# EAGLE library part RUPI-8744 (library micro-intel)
MICROCOMPUTER/PERIPHERAL DEVICE
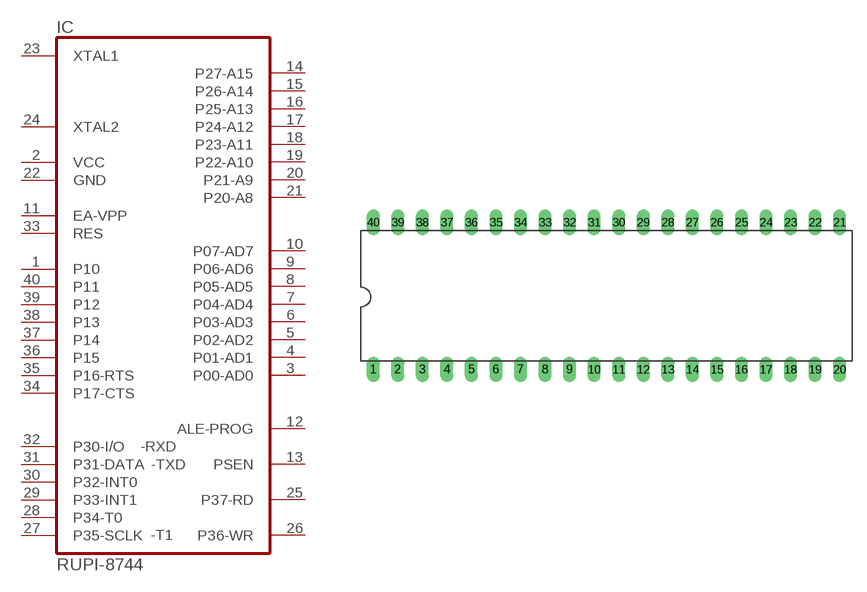
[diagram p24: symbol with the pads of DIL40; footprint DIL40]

Designator prefix IC

## RUPI-8744 (OC_FARNELL: unknown; OC_NEWARK: unknown)  [DIL40]
1  P10
2  VCC  pwr
3  P00-AD0
4  P01-AD1
5  P02-AD2
6  P03-AD3
7  P04-AD4
8  P05-AD5
9  P06-AD6
10  P07-AD7
11  EA-VPP  in
12  ALE-PROG  out
13  PSEN  out
14  P27-A15
15  P26-A14
16  P25-A13
17  P24-A12
18  P23-A11
19  P22-A10
20  P21-A9
21  P20-A8
22  GND  pwr
23  XTAL1  in
24  XTAL2  in
25  P37-RD
26  P36-WR
27  P35-SCLK
28  P34-T0
29  P33-INT1
30  P32-INT0
31  P31-DATA
32  P30-I/O
33  RES  in
34  P17-CTS
35  P16-RTS
36  P15
37  P14
38  P13
39  P12
40  P11

## Footprint DIL40 (pad centres in mm)
Dual In Line Package
drill 0.813 long: 1 -24.13,-7.62; 2 -21.59,-7.62; 3 -19.05,-7.62; 4 -16.51,-7.62; 5 -13.97,-7.62; 6 -11.43,-7.62; 7 -8.89,-7.62; 8 -6.35,-7.62; 9 -3.81,-7.62; 10 -1.27,-7.62; 11 1.27,-7.62; 12 3.81,-7.62; 13 6.35,-7.62; 14 8.89,-7.62; 15 11.43,-7.62; 16 13.97,-7.62; 17 16.51,-7.62; 18 19.05,-7.62; 19 21.59,-7.62; 20 24.13,-7.62; 21 24.13,7.62; 22 21.59,7.62; 23 19.05,7.62; 24 16.51,7.62; 25 13.97,7.62; 26 11.43,7.62; 27 8.89,7.62; 28 6.35,7.62; 29 3.81,7.62; 30 1.27,7.62; 31 -1.27,7.62; 32 -3.81,7.62; 33 -6.35,7.62; 34 -8.89,7.62; 35 -11.43,7.62; 36 -13.97,7.62; 37 -16.51,7.62; 38 -19.05,7.62; 39 -21.59,7.62; 40 -24.13,7.62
